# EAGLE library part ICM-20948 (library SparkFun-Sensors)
ICM-20948 9 Degree of Freedom IMU World’s lowest power 9-axis MotionTracking device that is ideally suited for smartphones, tablets, wearable sensors, and IoT applications. Includes onboard Digital Motion Processor to offload computations from the host processor Datasheet SparkFun Products: SparkFun IMU Breakout - ICM-20948
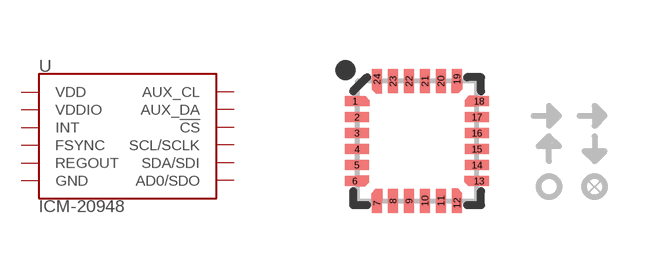
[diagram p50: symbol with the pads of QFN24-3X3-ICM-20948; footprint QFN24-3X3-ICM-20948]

Designator prefix U

## ICM-20948 (PROD_ID: IC-14247; VALUE: 9DoF IMU)  [QFN24-3X3-ICM-20948]
7  AUX_CL
8  VDDIO
9  AD0/SDO
10  REGOUT
11  FSYNC
12  INT
13  VDD
18  GND
20  GND
21  AUX_DA
22  !CS
23  SCL/SCLK
24  SDA/SDI

## Footprint QFN24-3X3-ICM-20948 (pad centres in mm)
24-Pin QFN - 3.0 x 3.0 mm - No center pad Note: No center pad per "Exposed Die Pad Precautions" section of the InvenSense MEMS Handling application note.
smd 0.495 x 0.25: 1 -1.552,1; 6 -1.552,-1; 13 1.552,-1; 18 1.552,1
smd 0.6 x 0.25: 2 -1.5,0.6; 3 -1.5,0.2; 4 -1.5,-0.2; 5 -1.5,-0.6; 14 1.5,-0.6; 15 1.5,-0.2; 16 1.5,0.2; 17 1.5,0.6
smd 0.25 x 0.495: 7 -1,-1.552; 12 1,-1.552; 19 1,1.552; 24 -1,1.552
smd 0.25 x 0.6: 8 -0.6,-1.5; 9 -0.2,-1.5; 10 0.2,-1.5; 11 0.6,-1.5; 20 0.6,1.5; 21 0.2,1.5; 22 -0.2,1.5; 23 -0.6,1.5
